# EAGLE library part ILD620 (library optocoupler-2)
SIEMENS OPTO COUPLER
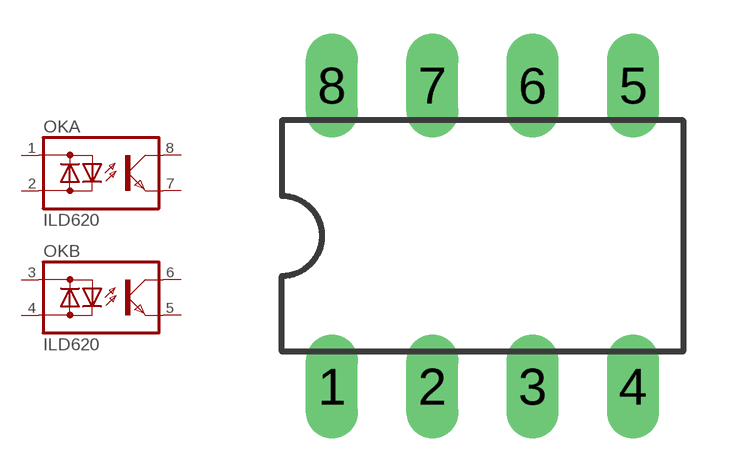
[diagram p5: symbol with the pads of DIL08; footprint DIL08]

Designator prefix OK; gates A=OK-LD B=OK-LD

## ILD620  [DIL08]
1  A:AC1  pas
2  A:AC2  pas
3  B:AC1  pas
4  B:AC2  pas
5  B:E  pas
6  B:C  pas
7  A:E  pas
8  A:C  pas

## Footprint DIL08 (pad centres in mm)
Dual In Line Package
drill 0.813 long: 1 -3.81,-3.81; 2 -1.27,-3.81; 3 1.27,-3.81; 4 3.81,-3.81; 5 3.81,3.81; 6 1.27,3.81; 7 -1.27,3.81; 8 -3.81,3.81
